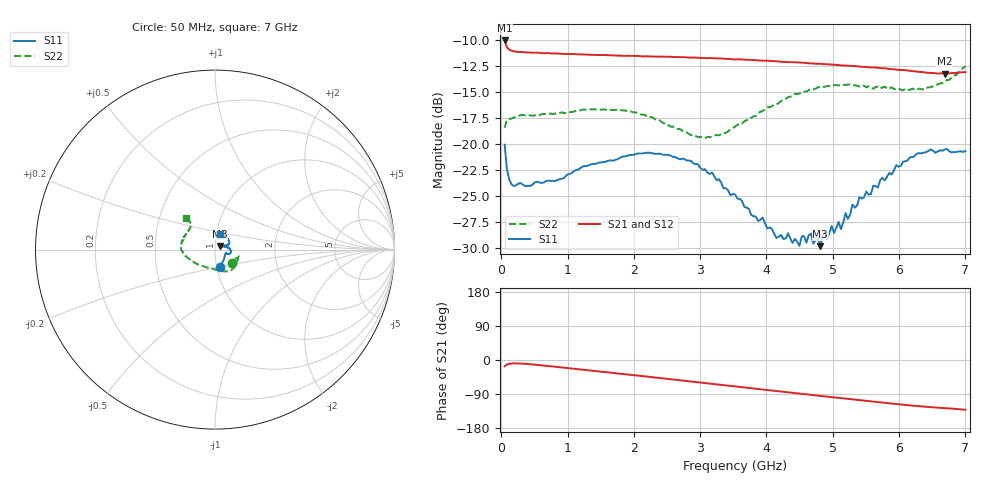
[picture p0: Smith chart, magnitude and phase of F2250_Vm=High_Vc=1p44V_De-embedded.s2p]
! Integrated Device Technology
! Corporate Headquarters
! 6024 Silver Creek Valley Road
! San Jose, CA 95138  USA
! Phone:  1-408-284-8200
! Toll Free:  1-800-223-1366
! Webpage:  http://www.idt.com/
! Timing and RF Division
! 515 Groton Road, Suite 102
! Westford, MA 01886-6024
! Device:  F2250
! Description: Voltage Variable RF Attenuator
! Frequency:  50.0 -  6000.00 MHz
! Package:  3x3 mm Thin QFN Plastic Package: 16 pin
! Ports:  2 RF, 3 DC
!  Pin  1  = GND
!  Pin  2  = NC
!  Pin  3  = RF1  = Port 1
!  Pin  4  = NC
!  Pin  5  = GND
!  Pin  6  = GND
!  Pin  7  = GND
!  Pin  8  = GND
!  Pin  9  = NC
!  Pin 10  = RF2  = Port 2
!  Pin 11  = NC
!  Pin 12  = GND
!  Pin 13  = GND
!  Pin 14  = VCNTRL
!  Pin 15  = VDD
!  Pin 16  = VMODE
! Vcntrl:  1.440 Volts
! Vmode:  +3.300 Volts
! Vdd:  +3.30  Volts
! Current:  1.331 mA
! Data:  The device was measured on a the F2250 evaluation board which has
!  individual transmission lines to the RF pins.  Data was collected
!  using a calibrated network analyzer.  The evaluation board was
!  de-embedded using a TRL calibration technique.
!  The reference plane is the edge of the package pin.
! Misc:  SN 10
!  Action Tracker AT0258
! Date Measured:  2014-11-26
! Date:  2015-10-15  MJV
! Note:
!  Integrated Device Technology supplies this data as a sample of measured
!  data at the package pin for this product.  Your particular data for this
!  product may vary.
!  Data was taken at 25 degrees C.
!  Integrated Device Technology reserves the right to change this data at anytime.
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# GHz S dB R 50
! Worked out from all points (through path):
!   201 points, 50 MHz to 7 GHz, reference 50 ohm
!   highest |S21| = -10.06 dB at 50 MHz (marker M1); lowest = -13.3 dB at 6.687 GHz (marker M2)
!   group delay of S21, straight-line fit = 52.1 ps
!   lowest |S11| = -29.8 dB at 4.811 GHz (marker M3), VSWR 1.07, Z = 52.6 + j2.06 ohm
!   |S11| at or under -10 dB: start of sweep to end of sweep
!   |S22| runs from -19.4 to -12.5 dB; largest |S21 - S12| = 0.0012
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0.05  -20.08 -73.9  -10.06 -16.6  -10.06 -16.6  -18.46 -37.1
0.1195  -23.45 -38.6  -10.95 -10.0  -10.95 -10.0  -17.60 -15.7
0.189  -24.04 -26.6  -11.11 -8.9  -11.11 -8.9  -17.48 -14.0
1.2315  -22.18 -19.0  -11.41 -25.6  -11.41 -25.6  -16.71 -41.7
2.37825  -20.94 -6.6  -11.62 -47.3  -11.63 -47.3  -17.68 -68.6
3.07325  -22.45 7.6  -11.76 -60.8  -11.76 -60.8  -19.45 -103.8
3.525  -24.87 19.9  -11.89 -69.7  -11.87 -69.8  -18.37 -133.1
4.1505  -29.07 38.8  -12.06 -81.9  -12.07 -81.9  -16.21 -161.2
4.32425  -28.61 39.7  -12.16 -85.2  -12.16 -85.3  -15.50 -166.9
4.498  -29.82 39.5  -12.19 -88.6  -12.18 -88.7  -15.18 -171.9
4.67175  -28.63 44.3  -12.27 -92.0  -12.27 -92.1  -14.75 -175.8
4.7065  -29.61 43.6  -12.27 -92.7  -12.27 -92.7  -14.77 -176.4
4.81075  -29.85 37.5  -12.31 -94.7  -12.29 -94.7  -14.52 -178.5
4.88025  -28.52 37.0  -12.34 -96.1  -12.34 -96.1  -14.51 179.4
4.915  -29.23 35.7  -12.35 -96.7  -12.35 -96.7  -14.46 178.6
4.9845  -27.93 34.4  -12.38 -98.1  -12.37 -98.1  -14.45 176.7
5.1235  -28.21 30.7  -12.46 -100.7  -12.45 -100.8  -14.35 173.8
5.29725  -25.85 22.7  -12.51 -104.0  -12.50 -104.1  -14.40 170.3
5.85325  -22.80 19.5  -12.81 -114.2  -12.80 -114.4  -14.69 155.1
6.27025  -20.93 26.5  -13.06 -121.4  -13.06 -121.5  -14.83 142.2
6.68725  -20.54 44.7  -13.26 -126.9  -13.25 -127.1  -13.99 132.1
7  -20.71 72.1  -13.10 -131.3  -13.10 -131.5  -12.52 132.6
